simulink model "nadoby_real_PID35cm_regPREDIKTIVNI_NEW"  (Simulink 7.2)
settings: Solver=ode15s  StartTime=0.0  StopTime=inf  RelTol=1e-3
undefined symbols (not defined in the file or in its folder): Humusoft, MF624, to, V
libraries: rtlib x3, simulink x2, mpclib x1

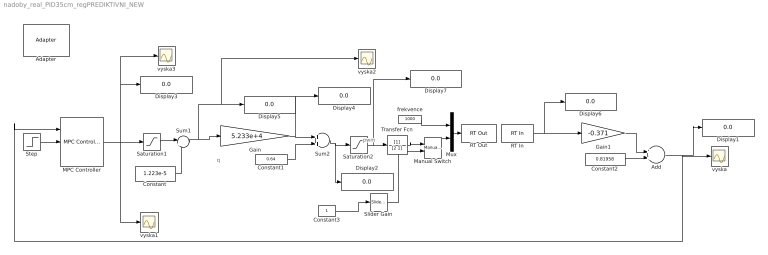
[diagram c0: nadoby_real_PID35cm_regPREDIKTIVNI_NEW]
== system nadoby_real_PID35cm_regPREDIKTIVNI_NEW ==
  note: pwm
  note: q
  Adapter : rtlib/Adapter  SystemSampleTime=-1  DriverName=Humusoft/MF624  DriverAddress=4294967295  DriverOptions=1
  Add : Sum  OutDataType=sfix(16)  OutScaling=2^-10
  Constant : Constant  Value=1.223e-5  OutDataType=fixdt(1, 16)  OutScaling=2^0
  Constant1 : Constant  Value=0.64  OutDataType=fixdt(1, 16)  OutScaling=2^0
  Constant2 : Constant  Value=0.81958  OutDataType=sfix(16)  OutScaling=2^0
  Constant3 : Constant  OutDataType=fixdt(1, 16)  OutScaling=2^0
  Display{1..7} (7 alike) : Display
  Gain : Gain  Gain=5.233e+4  ParameterDataType=sfix(16)  ParameterScaling=2^0  OutDataType=sfix(16)  OutScaling=2^0
  Gain1 : Gain  Gain=-0.371  ParameterDataType=sfix(16)  ParameterScaling=2^0  OutDataType=sfix(16)  OutScaling=2^0
  MPC Controller : mpclib/MPC Controller  SystemSampleTime=-1  mpcobj=mpc_controller  n_mv=0  x0=[]  ref_from_ws=off  ref_signal_name=[]  ref_preview=on  md_from_ws=off  md_signal_name=[]  md_preview=on  from_project=off  md_inport=on  mv_inport=off  lims_inport=off  switch_inport=off  enable_value=0  project_file=MPCtask.mat  is_multiple=0
  Manual Switch : simulink/Signal Routing/Manual Switch  SystemSampleTime=-1  sw=0  action=0  varsize=off
  Mux : Mux  Inputs=2
  RT In : rtlib/RT In  SampleTime=0.01  Adapter=Adapter  IOClass=Analog Input  Channels=1  SLDataType=double  MaxMissedTicks=inf  ShowMissedTicks=off  YieldWhenWaiting=on  AIORange=-10 to 10 V  AIOUnits=Volts  DIOMode=Bit  CIReset=never  CIEdge=rising  CIGate=none  EIQuadrature=quadruple  EIIndexPulse=reset  EIFilterFrequency=Inf  OIOParameters=[]
  RT Out : rtlib/RT Out  SampleTime=0.1  Adapter=Adapter  IOClass=Other Output  Channels=[1 2]  InitialValue=[]  FinalValue=[]  MaxMissedTicks=inf  ShowMissedTicks=off  YieldWhenWaiting=on  AIORange=-10 to 10 V  AIOUnits=Volts  DIOMode=Bit  OIOParameters=[]
  Saturation1 : Saturate  UpperLimit=1.9109e-5  LowerLimit=0  ZeroCross=off  OutDataType=fixdt(1, 16)  OutScaling=2^0
  Saturation2 : Saturate  UpperLimit=1  LowerLimit=0.445  ZeroCross=off  OutDataType=fixdt(1, 16)  OutScaling=2^0
  Slider Gain : simulink/Math Operations/Slider Gain  SystemSampleTime=-1  low=0  gain=0.31797  high=1
  Step : Step  Time=0  After=0.35  SampleTime=0
  Sum1 : Sum  Inputs=|+-  OutDataType=fixdt(1, 16)  OutScaling=2^0
  Sum2 : Sum  OutDataType=fixdt(1, 16)  OutScaling=2^0
  Transfer Fcn : TransferFcn  Denominator=[2 1]
  frekvence : Constant  Value=1000  OutDataType=fixdt(1, 16)  OutScaling=2^0
  vyska{,1..3} (4 alike) : Scope
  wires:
  Sum1/1 -> Gain/1, Display5/1, vyska2/1
  MPC Controller/1 -> vyska1/1, Display3/1, vyska3/1, Saturation1/1
  frekvence/1 -> Mux/1
  Gain1/1 -> Add/1
  Constant2/1 -> Add/2
  RT In/1 -> Gain1/1, Display6/1
  Add/1 -> vyska/1, Display1/1, MPC Controller/1
  Step/1 -> MPC Controller/2
  Gain/1 -> Sum2/1, Display4/1
  Sum2/1 -> Display2/1, Saturation2/1
  Mux/1 -> RT Out/1
  Manual Switch/1 -> Mux/2
  Constant3/1 -> Slider Gain/1
  Constant1/1 -> Sum2/2
  Slider Gain/1 -> Manual Switch/2
  Saturation2/1 -> Transfer Fcn/1, Display7/1
  Transfer Fcn/1 -> Manual Switch/1
  Saturation1/1 -> Sum1/1
  Constant/1 -> Sum1/2
